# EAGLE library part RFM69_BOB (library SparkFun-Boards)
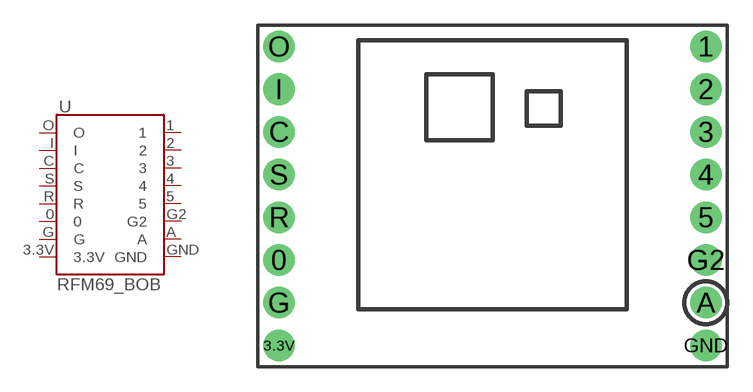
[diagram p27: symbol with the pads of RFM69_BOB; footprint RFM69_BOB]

Designator prefix -

## RFM69_BOB  [RFM69_BOB]
0  0
1  1
2  2
3  3
3.3V  3.3V
4  4
5  5
A  A
C  C
G  G
G2  G2
GND  GND
I  I
O  O
R  R
S  S

## Footprint RFM69_BOB (pad centres in mm)
drill 1.118 pad 1.88: 0 -12.7,-3.81; 1 12.7,8.89; 2 12.7,6.35; 3 12.7,3.81; 3.3V -12.7,-8.89; 4 12.7,1.27; 5 12.7,-1.27; A 12.7,-6.35; C -12.7,3.81; G -12.7,-6.35; G2 12.7,-3.81; GND 12.7,-8.89; I -12.7,6.35; O -12.7,8.89; R -12.7,-1.27; S -12.7,1.27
